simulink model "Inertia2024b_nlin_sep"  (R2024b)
settings: Solver=ode1  StartTime=0.0  StopTime=30  FixedStep=Tstep  EnableMultiTasking=on
model workspace (MAT data in the model file):
  op_snapshot1 : opcond.OperatingPoint (value not decoded)
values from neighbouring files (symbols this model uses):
  T_dis = 2.5    [onebus_nonlinsub.m]
  Ts = Tstep    (= 1e-05)    [onebus_nonlinsub.m]    (also in DemoMTI_Boolean_Index_MTI.m = 1; DemoMTI_EKF.m = 0.02; DemoMTI_MHE_VanDePol.m = 0.01)
  Tstep = 1e-5    (= 1e-05)    [DemoMTI_greyestGFM.m]    (also in onebus_nonlinsub.m)
  Vn = 380    [simulink_parameters_one_bus.m]    (also in nine_bus_parameters.m = 310.*ones(num_inv,1))
  Vtri = Vdc1./3    [simulink_parameters_one_bus.m]    (also in nine_bus_parameters.m = Vdc./2)
  wn = ones(num_inv,1).*w01    [nine_bus_parameters.m]    (also in computeModeFrequencyDampingTable.m = abs(lambda))
undefined symbols (not defined in the file or in its folder): D1_g1, Dsg, Dxd, Dxq, Efdmax_g1, Efdmin_g1, Ibg, K_int_pll, K_prop_pll, KA_g1, kpss_g1, L_1_2, M1_g1, Msg, nom, op, R_1_2, ra_g1, Rsg, T1_g1, T2_g1, T3_g1, T4_g1, TA_g1, Td, Td0p_g1, Tq0p_g1, Tv, Tw_g1, Vbg, xdp_g1, xqp_g1
libraries: spsThreePhaseVIMeasurementLib x5, spsGroundLib x4, slpidlib x4, spsControlledVoltageSourceLib x3, spsControlledCurrentSourceLib x3, spsSeriesRLCBranchLib x3, spsThreePhaseSeriesRLCBranchLib x2, spsThreePhaseSeriesRLCLoadLib x2, spsThreePhaseTransformerTwoWindingsLib x1, spsThreePhaseDynamicLoadLib x1, spsSampleandHoldLib x1, sps_lib x1
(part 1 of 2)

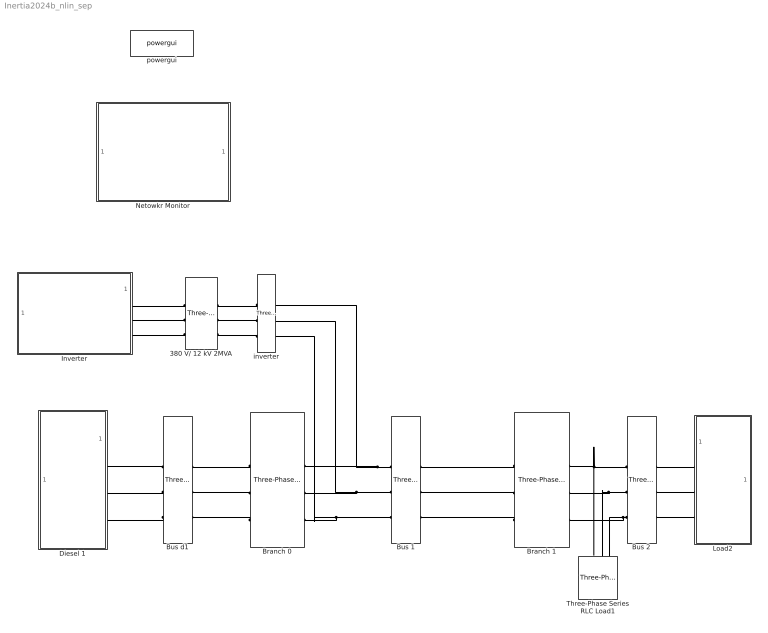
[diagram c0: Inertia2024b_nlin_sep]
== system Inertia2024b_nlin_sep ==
  380 V/ 12 kV 2MVA : spsThreePhaseTransformerTwoWindingsLib/Three-Phase Transformer (Two Windings)  Winding1Connection=Yg  Winding2Connection=Yg  CoreType=Three single-phase transformers  SetSaturation=off  Hysteresis=off  DataFile='hysteresis'  SetInitialFlux=off  Measurements=None  UNITS=pu  NominalPower="[2e6  60]"  Winding1=[12.66e3 , 0.025/30 , 0.025]  Winding2=[380, 0.025/30 , 0.025]  Rm=500  Lm=inf  L0=0.5  Saturation=[ 0,0 ; 0.0024,1.2 ; 1.0,1.52 ]  InitialFluxes=[ 0.8 , -0.8 , 0.7 ]  BreakLoop=off  DiscreteSolver=Trapezoidal iterative  DataType=off  TransfoNumber=0
  Branch 0 : spsThreePhaseSeriesRLCBranchLib/Three-Phase Series RLC Branch  LConnTagsString=A|B|C  RConnTagsString=A|B|C  BranchType=RL  Resistance=0.05  Inductance=0.1/(nom.W)  Capacitance=1e-6  Measurements=None
  Branch 1 : spsThreePhaseSeriesRLCBranchLib/Three-Phase Series RLC Branch  LConnTagsString=A|B|C  RConnTagsString=A|B|C  BranchType=RL  Resistance=R_1_2  Inductance=L_1_2  Capacitance=1e-6  Measurements=None
  Bus 1 : spsThreePhaseVIMeasurementLib/Three-Phase V-I Measurement  VoltageMeasurement=phase-to-ground  SetLabelV=on  LabelV=Vabc1  Vpu=off  VpuLL=off  CurrentMeasurement=yes  SetLabelI=on  LabelI=Iabc1  Ipu=off  Pbase=100e6  Vbase=500e3  OutputType=Complex  PhasorSimulation=off  PSBequivalent=0
  Bus 2 : spsThreePhaseVIMeasurementLib/Three-Phase V-I Measurement  VoltageMeasurement=phase-to-ground  SetLabelV=on  LabelV=Vabc2  Vpu=off  VpuLL=off  CurrentMeasurement=yes  SetLabelI=on  LabelI=Iabc2  Ipu=off  Pbase=100e6  Vbase=500e3  OutputType=Complex  PhasorSimulation=off  PSBequivalent=0
  Bus d1 : spsThreePhaseVIMeasurementLib/Three-Phase V-I Measurement  VoltageMeasurement=phase-to-ground  SetLabelV=on  LabelV=Vabc_d1  Vpu=off  VpuLL=off  CurrentMeasurement=yes  SetLabelI=on  LabelI=Iabc_d1  Ipu=off  Pbase=100e6  Vbase=500e3  OutputType=Complex  PhasorSimulation=off  PSBequivalent=0
  Diesel 1 : Subsystem
  Inverter : Subsystem
  Load2 : Subsystem
  Netowkr Monitor : Subsystem
  Three-Phase Series RLC Load1 : spsThreePhaseSeriesRLCLoadLib/Three-Phase Series RLC Load  LConnTagsString=A|B|C  Configuration=Y (grounded)  NominalVoltage=Vn_pp  Vabc=[1e3 1e3 1e3]  Vabcp=[1e3 1e3 1e3]  NominalFrequency=60  UnbalancedPower=off  ActivePower=P2  InductivePower=Q2  CapacitivePower=0  Pabc=[10e3 9e3 11e3]  QLabc=[100 90 110]  QCabc=[100 90 110]  Pabcp=[10e3 9e3 11e3]  QLabcp=[100 90 110]  QCabcp=[100 90 110]  Measurements=None  LoadType=constant PQ
  inverter : spsThreePhaseVIMeasurementLib/Three-Phase V-I Measurement  VoltageMeasurement=phase-to-ground  SetLabelV=on  LabelV=Vabc_inverter  Vpu=off  VpuLL=off  CurrentMeasurement=yes  SetLabelI=on  LabelI=Iabc_inverter  Ipu=off  Pbase=100e6  Vbase=500e3  OutputType=Complex  PhasorSimulation=off  PSBequivalent=0
  powergui : sps_lib/powergui  Priority=1  SimulationMode=Discrete  SampleTime=Tstep  frequency=60  Iterations=50  frequencyindice=0  Pbase=100e6  ErrMax=1e-4  UnitsV=kV  UnitsW=MW  buscounter=0  FunctionMessages=off  echomessages=off  EnableUseOfTLC=on  CurrentSourceSwitches=off  DisableSnubberDevices=off  DisableRonSwitches=off  DisableVfSwitches=off  DisplayEquations=off  AutomaticDiscreteSolvers=off  SolverType=Tustin/Backward Euler (TBE)  Interpol=off  ExternalGateDelay=off  methode=off  Ts=0  x0status=blocks  SPID=off  SwTol=0  HookPort=off  NonlinearTolerance=1e-4  nMaxIteration=100  ContinueOnMaxIteration=off  RestoreLinks=warning  ResistiveCurrentMeasurement=off  Frange=[0:2:500]  Ylog=off  Xlog=on  ShowGrid=off  save=off  variable=ZData  structure=0  ZoomFFT=on  StartTime=0.0  cycles=1  DisplayStyle=1  fundamental=60  FreqAxis=off  MaxFrequency=1000  frequencyindicesteady=1  RmsSteady=1  display=off
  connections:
  Branch 1/LConn1 -- Bus 1/RConn1
  Branch 1/LConn2 -- Bus 1/RConn2
  Branch 1/LConn3 -- Bus 1/RConn3
  Bus 2/LConn1 -- Three-Phase Series RLC Load1/LConn1 -- Branch 1/RConn1
  Bus 2/LConn2 -- Three-Phase Series RLC Load1/LConn2 -- Branch 1/RConn2
  Bus 2/LConn3 -- Three-Phase Series RLC Load1/LConn3 -- Branch 1/RConn3
  Bus 1/LConn1 -- inverter/RConn1 -- Branch 0/RConn1
  Bus 1/LConn2 -- inverter/RConn2 -- Branch 0/RConn2
  Bus 1/LConn3 -- inverter/RConn3 -- Branch 0/RConn3
  Branch 0/LConn1 -- Bus d1/RConn1
  Bus d1/LConn1 -- Diesel 1/RConn1
  Branch 0/LConn3 -- Bus d1/RConn3
  Bus d1/LConn3 -- Diesel 1/RConn3
  Bus d1/LConn2 -- Diesel 1/RConn2
  Branch 0/LConn2 -- Bus d1/RConn2
  Bus 2/RConn3 -- Load2/LConn3
  Bus 2/RConn2 -- Load2/LConn2
  Bus 2/RConn1 -- Load2/LConn1
  Inverter/RConn2 -- 380 V/ 12 kV 2MVA/RConn2
  inverter/LConn2 -- 380 V/ 12 kV 2MVA/LConn2
  inverter/LConn1 -- 380 V/ 12 kV 2MVA/LConn1
  Inverter/RConn1 -- 380 V/ 12 kV 2MVA/RConn1
  Inverter/RConn3 -- 380 V/ 12 kV 2MVA/RConn3
  inverter/LConn3 -- 380 V/ 12 kV 2MVA/LConn3

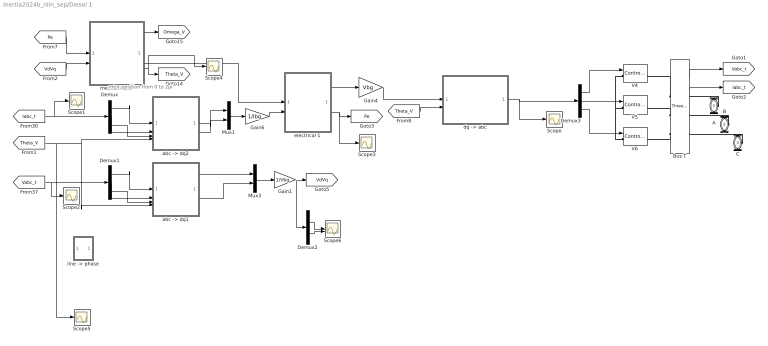
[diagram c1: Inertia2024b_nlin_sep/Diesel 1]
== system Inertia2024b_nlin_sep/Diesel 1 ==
  note: rotor position from 0 to 2pi
  Bus T : spsThreePhaseVIMeasurementLib/Three-Phase V-I Measurement  VoltageMeasurement=phase-to-ground  SetLabelV=off  LabelV=Vabc_d1  Vpu=off  VpuLL=off  CurrentMeasurement=yes  SetLabelI=off  LabelI=Iabc_d1  Ipu=off  Pbase=100e6  Vbase=500e3  OutputType=Complex  PhasorSimulation=off  PSBequivalent=0
  Demux : Demux  Outputs=3
  Demux1 : Demux  Outputs=3
  Demux2 : Demux  Outputs=2
  Demux3 : Demux  Outputs=3
  Gain1 : Gain  Gain=1/Vbg
  Gain4 : Gain  Gain=Vbg
  Gain6 : Gain  Gain=1/Ibg
  Mux1 : Mux  Inputs=2
  Mux3 : Mux  Inputs=2
  Scope{,1..5} (6 alike) : Scope
  Scope6 : Scope  NumInputPorts=2
  V4 : spsControlledVoltageSourceLib/Controlled Voltage Source  Initialize=off  Source_Type=AC  Amplitude=Vbg  Phase=0  Frequency=60  Measurements=None
  V5 : spsControlledVoltageSourceLib/Controlled Voltage Source  Initialize=off  Source_Type=AC  Amplitude=Vbg  Phase=-120  Frequency=60  Measurements=None
  V6 : spsControlledVoltageSourceLib/Controlled Voltage Source  Initialize=off  Source_Type=AC  Amplitude=Vbg  Phase=120  Frequency=60  Measurements=None
  "abc -> dq1" : Subsystem
  "abc -> dq2" : Subsystem
  "dq -> abc" : Subsystem
  electrical 1 : Subsystem
  "line -> phase" : Subsystem  Commented=on
  mechanical 1 : Subsystem
  A : PMIOPort  Side=Right
  B : PMIOPort  Port=2  Side=Right
  C : PMIOPort  Port=3  Side=Right
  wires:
  "abc -> dq2"/1(d) -> Mux1/1
  "abc -> dq1"/1(d) -> Mux3/1
  [Theta_V] -> Scope5/1, "abc -> dq2"/4(Theta), "abc -> dq1"/4(Theta)
  "abc -> dq2"/2(q) -> Mux1/2
  Mux1/1 -> Gain6/1
  electrical 1/2(Pe) -> Scope3/1, [Pe]
  mechanical 1/2(Ef) -> electrical 1/1(Efd)
  electrical 1/1(VdVqref) -> Gain4/1
  Gain6/1 -> electrical 1/2(IdIq)
  Gain4/1 -> "dq -> abc"/1(dq)
  [Theta_V] -> "dq -> abc"/2(Theta)
  Mux3/1 -> Gain1/1
  Gain1/1 -> Demux2/1, [VdVq]
  Demux3/1 -> V4/1
  Demux3/2 -> V5/1
  Demux3/3 -> V6/1
  "dq -> abc"/1(abc) -> Demux3/1, Scope/1
  [Iabc_t] -> Scope1/1, Demux/1
  Demux/1 -> "abc -> dq2"/1(a)
  Demux/2 -> "abc -> dq2"/2(b)
  Demux/3 -> "abc -> dq2"/3(c)
  "abc -> dq1"/2(q) -> Mux3/2
  Demux1/2 -> "abc -> dq1"/2(b)
  Demux1/1 -> "abc -> dq1"/1(a)
  Demux1/3 -> "abc -> dq1"/3(c)
  [Vabc_t] -> Scope2/1, Demux1/1
  mechanical 1/1(w) -> [Omega_V]
  [Pe] -> mechanical 1/1(Pe)
  [VdVq] -> mechanical 1/2(VdVqFB)
  Bus T/1 -> [Vabc_t]
  Bus T/2 -> [Iabc_t]
  mechanical 1/3(rotor angle) -> Scope4/1, [Theta_V]
  Demux2/1 -> Scope6/1
  Demux2/2 -> Scope6/2
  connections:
  V5/LConn1 -- V4/LConn1 -- V6/LConn1
  Bus T/LConn1 -- V4/RConn1
  Bus T/LConn2 -- V5/RConn1
  Bus T/LConn3 -- V6/RConn1
  C/RConn1 -- Bus T/RConn3
  B/RConn1 -- Bus T/RConn2
  A/RConn1 -- Bus T/RConn1

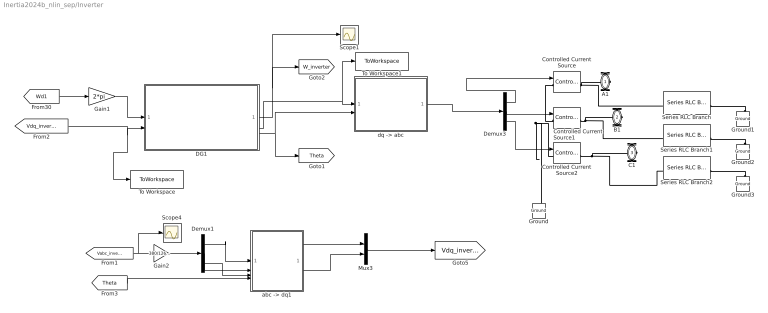
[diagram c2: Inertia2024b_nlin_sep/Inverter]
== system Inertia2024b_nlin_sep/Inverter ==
  Controlled Current Source : spsControlledCurrentSourceLib/Controlled Current Source  Initialize=off  Source_Type=AC  Amplitude=0  Phase=0  Frequency=0  Measurements=None
  Controlled Current Source1 : spsControlledCurrentSourceLib/Controlled Current Source  Initialize=off  Source_Type=AC  Amplitude=0  Phase=0  Frequency=0  Measurements=None
  Controlled Current Source2 : spsControlledCurrentSourceLib/Controlled Current Source  Initialize=off  Source_Type=AC  Amplitude=0  Phase=0  Frequency=0  Measurements=None
  DG1 : Subsystem  ReferencedSubsystem=inverter_nonlinear_model2024b  rdc=rdc1  Ldc=Ldc1  Cdc=Cdc1  Vdc=Vdc1  Cf=Cf1  Lf=Lf1  rf=rf1  rc=rc1  Lc=Lc1  wc=wc1  mp=mp1  nq=nq1  Vn=Vn(1)  wn=wn(1)  Kic=Kic1  Kpc=Kpc1  Kiv=Kiv1  Kpv=Kpv1  F=F1  Vtri=Vtri(1)  x0=x01
  Demux1 : Demux  Outputs=3
  Demux3 : Demux  Outputs=3
  Gain1 : Gain  Gain=2*pi
  Gain2 : Gain  Gain=380/12600
  Ground{,1..3} (4 alike) : spsGroundLib/Ground  LConnTagsString=a
  Mux3 : Mux  Inputs=2
  Scope1 : Scope
  Scope4 : Scope
  Series RLC Branch : spsSeriesRLCBranchLib/Series RLC Branch  LConnTagsString=__new0  RConnTagsString=__new0  BranchType=RLC  Resistance=1e6  Inductance=0  SetiL0=off  InitialCurrent=0  Capacitance=0  Setx0=off  InitialVoltage=0  Measurements=None
  Series RLC Branch1 : spsSeriesRLCBranchLib/Series RLC Branch  LConnTagsString=__new0  RConnTagsString=__new0  BranchType=RLC  Resistance=1e6  Inductance=0  SetiL0=off  InitialCurrent=0  Capacitance=0  Setx0=off  InitialVoltage=0  Measurements=None
  Series RLC Branch2 : spsSeriesRLCBranchLib/Series RLC Branch  LConnTagsString=__new0  RConnTagsString=__new0  BranchType=RLC  Resistance=1e6  Inductance=0  SetiL0=off  InitialCurrent=0  Capacitance=0  Setx0=off  InitialVoltage=0  Measurements=None
  To Workspace : ToWorkspace  VariableName=Vdq_inv  SaveFormat=Timeseries  SampleTime=-1
  To Workspace1 : ToWorkspace  VariableName=ioDQ  SaveFormat=Timeseries  SampleTime=-1
  "abc -> dq1" : Subsystem
  "dq -> abc" : Subsystem
  A1 : PMIOPort  Side=Right
  B1 : PMIOPort  Port=2  Side=Right
  C1 : PMIOPort  Port=3  Side=Right
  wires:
  [Wd1] -> Gain1/1
  DG1/2 -> To Workspace1/1, "dq -> abc"/1(dq)
  "dq -> abc"/1(abc) -> Demux3/1
  Demux3/3 -> Controlled Current Source2/1
  Demux3/2 -> Controlled Current Source1/1
  Demux3/1 -> Controlled Current Source/1
  Gain1/1 -> DG1/1
  [Vdq_inverter] -> To Workspace/1, DG1/2
  Demux1/2 -> "abc -> dq1"/2(b)
  "abc -> dq1"/1(d) -> Mux3/1
  [Theta] -> "abc -> dq1"/4(Theta)
  [Vabc_inverter] -> Scope4/1, Gain2/1
  Mux3/1 -> [Vdq_inverter]
  "abc -> dq1"/2(q) -> Mux3/2
  Demux1/1 -> "abc -> dq1"/1(a)
  Demux1/3 -> "abc -> dq1"/3(c)
  DG1/3 -> "dq -> abc"/2(Theta), [Theta]
  DG1/1 -> [W_inverter], Scope1/1
  Gain2/1 -> Demux1/1
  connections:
  Controlled Current Source/LConn1 -- Ground/LConn1 -- Controlled Current Source2/LConn1 -- Controlled Current Source1/LConn1
  Controlled Current Source/RConn1 -- Series RLC Branch/LConn1 -- A1/RConn1
  Controlled Current Source1/RConn1 -- Series RLC Branch1/LConn1 -- B1/RConn1
  Controlled Current Source2/RConn1 -- Series RLC Branch2/LConn1 -- C1/RConn1
  Ground1/LConn1 -- Series RLC Branch/RConn1
  Ground2/LConn1 -- Series RLC Branch1/RConn1
  Ground3/LConn1 -- Series RLC Branch2/RConn1

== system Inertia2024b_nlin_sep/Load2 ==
  Bus Selector2 : BusSelector  OutputSignals=Positive-sequence voltage V (pu),Active power P (W),Reactive power Q (var)
  P3 : spsThreePhaseDynamicLoadLib/Three-Phase Dynamic Load  NominalVoltage=[nom.V nom.F]  ActiveReactivePowers="[op.PL1  op.QL1]"  PositiveSequence=[1 0]  ExternalControl=on  NpNq=[0 0]  TimeConstants="[0  0  0  0]"  MinimumVoltage=0.7  Tfilter=1e-4  LoadFlowParameters=[4,0,0,0,0]
  PQref3 : Subsystem
  Three-Phase Series RLC Load : spsThreePhaseSeriesRLCLoadLib/Three-Phase Series RLC Load  LConnTagsString=A|B|C  Configuration=Y (grounded)  NominalVoltage=nom.V  Vabc=[1e3 1e3 1e3]  Vabcp=[1e3 1e3 1e3]  NominalFrequency=nom.F  UnbalancedPower=off  ActivePower=10e3  InductivePower=0  CapacitivePower=0  Pabc=[10e3 9e3 11e3]  QLabc=[100 90 110]  QCabc=[100 90 110]  Pabcp=[10e3 9e3 11e3]  QLabcp=[100 90 110]  QCabcp=[100 90 110]  Measurements=None  LoadType=constant PQ
  scope7 : Scope
  A : PMIOPort  Side=Left
  B : PMIOPort  Port=2  Side=Left
  C : PMIOPort  Port=3  Side=Left
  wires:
  P3/1 -> scope7/1, Bus Selector2/1
  Bus Selector2/1 -> PQref3/1(V), [V_Load10]  "<Positive-sequence voltage V (pu)>"
  Bus Selector2/2 -> [P_Load10]  "<Active power P (W)>"
  Bus Selector2/3 -> [Q_Load10]  "<Reactive power Q (var)>"
  PQref3/1(PQ) -> P3/1
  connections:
  C/RConn1 -- Three-Phase Series RLC Load/LConn3 -- P3/LConn3
  B/RConn1 -- Three-Phase Series RLC Load/LConn2 -- P3/LConn2
  A/RConn1 -- Three-Phase Series RLC Load/LConn1 -- P3/LConn1

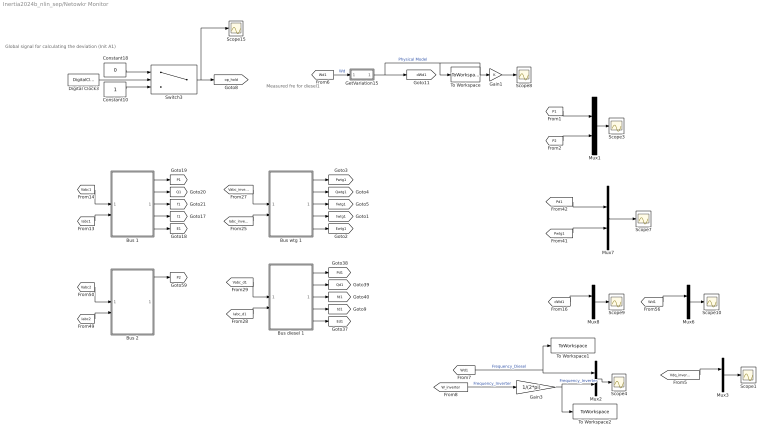
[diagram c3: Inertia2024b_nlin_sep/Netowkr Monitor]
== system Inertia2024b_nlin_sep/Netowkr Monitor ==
  note: Global signal for calculating the deviation (Init A1)
  note: Measured fre for diesel1
  Bus 1 : Subsystem
  Bus 2 : Subsystem
  Bus diesel 1 : Subsystem
  Bus wtg 1 : Subsystem
  Constant10 : Constant
  Constant18 : Constant  Value=0
  Digital Clock3 : DigitalClock  SampleTime=Ts
  Gain1 : Gain
  Gain3 : Gain  Gain=1/(2*pi)
  GetVariation15 : Subsystem
  Mux1 : Mux  Inputs=2
  Mux2 : Mux  Inputs=2
  Mux3 : Mux  Inputs=1
  Mux6 : Mux  Inputs=1
  Mux7 : Mux  Inputs=2
  Mux8 : Mux  Inputs=1
  Scope{1,3..4,7..10,15} (8 alike) : Scope
  Switch3 : Switch  Threshold=T_dis
  To Workspace : ToWorkspace  VariableName=y_con  SaveFormat=Structure With Time  SampleTime=-1
  To Workspace1 : ToWorkspace  VariableName=Wd1  SaveFormat=Timeseries  SampleTime=-1
  To Workspace2 : ToWorkspace  VariableName=W_inverter  SaveFormat=Timeseries  SampleTime=-1
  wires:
  [Vabc1] -> Bus 1/1(Vabc)
  [Iabc1] -> Bus 1/2(I_abc)
  Bus 1/1(P_meas) -> [P1]
  Bus 1/2(Q_meas) -> [Q1]
  Bus 1/3(w_meas) -> [f1]
  Bus 1/4(theta) -> [t1]
  Bus 1/5(E) -> [E1]
  Mux1/1 -> Scope3/1
  [P2] -> Mux1/2
  [P1] -> Mux1/1
  [Vabc_inverter] -> Bus wtg 1/1(Vabc)
  [Iabc_inverter] -> Bus wtg 1/2(I_abc)
  Bus wtg 1/1(P_meas) -> [Pwtg1]
  Bus wtg 1/2(Q_meas) -> [Qwtg1]
  Bus wtg 1/3(w_meas) -> [fwtg1]
  Bus wtg 1/4(theta) -> [twtg1]
  Bus wtg 1/5(E) -> [Ewtg1]
  [Pd1] -> Mux7/1
  Mux7/1 -> Scope7/1
  [Pwtg1] -> Mux7/2
  [Vabc2] -> Bus 2/1(Vabc)
  [Iabc2] -> Bus 2/2(I_abc)
  Bus 2/1(P_meas) -> [P2]
  [Wd1] -> Mux6/1
  Mux6/1 -> Scope10/1
  Switch3/1 -> [op_hold], Scope15/1
  Constant10/1 -> Switch3/3
  Digital Clock3/1 -> Switch3/2
  Constant18/1 -> Switch3/1
  [Wd1] -> GetVariation15/1(In1)  "Wd"
  GetVariation15/1(Out1) -> Gain1/1, To Workspace/1, [dWd1]  "Physical Model"
  Gain1/1 -> Scope8/1
  Mux8/1 -> Scope9/1
  [dWd1] -> Mux8/1
  Bus diesel 1/4(theta) -> [td1]
  Bus diesel 1/3(w_meas) -> [fd1]
  [Vabc_d1] -> Bus diesel 1/1(Vabc)
  Bus diesel 1/5(E) -> [Ed1]
  Bus diesel 1/2(Q_meas) -> [Qd1]
  [Iabc_d1] -> Bus diesel 1/2(I_abc)
  Bus diesel 1/1(P_meas) -> [Pd1]
  Mux3/1 -> Scope1/1
  [Vdq_inverter] -> Mux3/1
  Gain3/1 -> To Workspace2/1, Mux2/2  "Frequency_Inverter"
  [W_inverter] -> Gain3/1  "Frequency_Inverter"
  [Wd1] -> To Workspace1/1, Mux2/1  "Frequency_Diesel"
  Mux2/1 -> Scope4/1

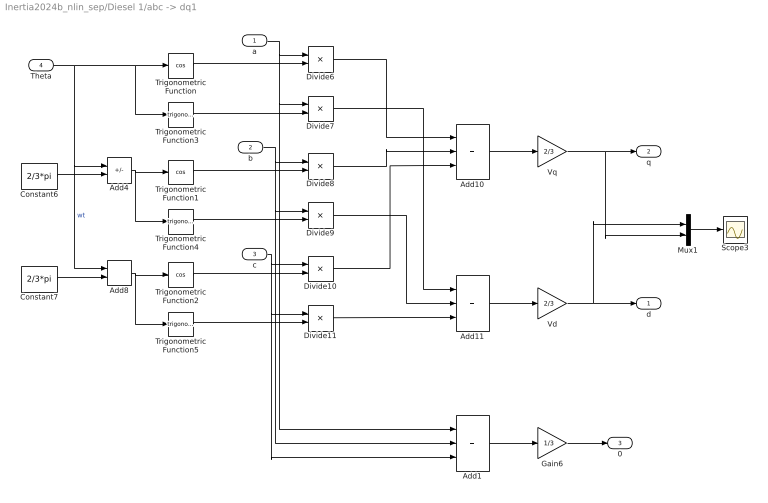
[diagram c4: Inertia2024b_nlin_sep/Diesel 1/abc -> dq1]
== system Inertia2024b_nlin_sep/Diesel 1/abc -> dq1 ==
  a : Inport
  b : Inport  Port=2
  c : Inport  Port=3
  Theta : Inport  Port=4
  Add1 : Sum  Inputs=+++
  Add10 : Sum  Inputs=+++
  Add11 : Sum  Inputs=+++
  Add4 : Sum  Inputs=+-
  Add8 : Sum
  Constant6 : Constant  Value=2/3*pi
  Constant7 : Constant  Value=2/3*pi
  Divide{6..11} (6 alike) : Product  Inputs=**
  Gain6 : Gain  Gain=1/3
  Mux1 : Mux  Inputs=2
  Scope3 : Scope
  Trigonometric Function : Trigonometry  Operator=cos
  Trigonometric Function1 : Trigonometry  Operator=cos
  Trigonometric Function2 : Trigonometry  Operator=cos
  Trigonometric Function3 : Trigonometry
  Trigonometric Function4 : Trigonometry
  Trigonometric Function5 : Trigonometry
  Vd : Gain  Gain=2/3
  Vq : Gain  Gain=2/3
  d : Outport  VectorParamsAs1DForOutWhenUnconnected=off
  q : Outport  Port=2  VectorParamsAs1DForOutWhenUnconnected=off
  0 : Outport  Port=3  VectorParamsAs1DForOutWhenUnconnected=off
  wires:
  Theta/1 -> Add4/1, Add8/1, Trigonometric Function/1, Trigonometric Function3/1  "wt"
  Constant6/1 -> Add4/2
  Add4/1 -> Trigonometric Function1/1, Trigonometric Function4/1
  Add8/1 -> Trigonometric Function2/1, Trigonometric Function5/1
  Trigonometric Function3/1 -> Divide7/2
  Trigonometric Function4/1 -> Divide9/2
  Trigonometric Function5/1 -> Divide11/2
  a/1 -> Divide6/1, Divide7/1, Add1/1
  Trigonometric Function/1 -> Divide6/2
  Trigonometric Function2/1 -> Divide10/2
  Trigonometric Function1/1 -> Divide8/2
  b/1 -> Divide8/1, Divide9/1, Add1/2
  c/1 -> Divide10/1, Divide11/1, Add1/3
  Constant7/1 -> Add8/2
  Divide6/1 -> Add10/1
  Divide8/1 -> Add10/2
  Divide10/1 -> Add10/3
  Divide7/1 -> Add11/1
  Divide9/1 -> Add11/2
  Divide11/1 -> Add11/3
  Add10/1 -> Vq/1
  Add11/1 -> Vd/1
  Vq/1 -> Mux1/2, q/1
  Vd/1 -> Mux1/1, d/1
  Add1/1 -> Gain6/1
  Gain6/1 -> 0/1
  Mux1/1 -> Scope3/1

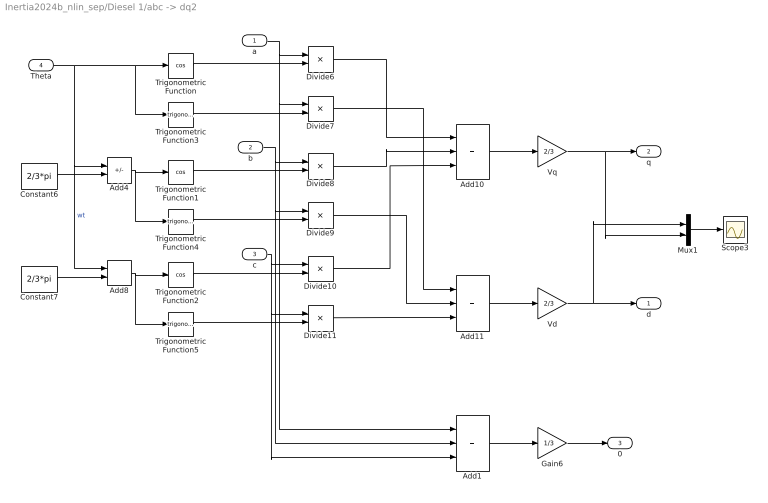
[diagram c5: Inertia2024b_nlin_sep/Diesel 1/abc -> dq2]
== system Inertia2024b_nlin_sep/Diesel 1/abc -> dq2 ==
  a : Inport
  b : Inport  Port=2
  c : Inport  Port=3
  Theta : Inport  Port=4
  Add1 : Sum  Inputs=+++
  Add10 : Sum  Inputs=+++
  Add11 : Sum  Inputs=+++
  Add4 : Sum  Inputs=+-
  Add8 : Sum
  Constant6 : Constant  Value=2/3*pi
  Constant7 : Constant  Value=2/3*pi
  Divide{6..11} (6 alike) : Product  Inputs=**
  Gain6 : Gain  Gain=1/3
  Mux1 : Mux  Inputs=2
  Scope3 : Scope
  Trigonometric Function : Trigonometry  Operator=cos
  Trigonometric Function1 : Trigonometry  Operator=cos
  Trigonometric Function2 : Trigonometry  Operator=cos
  Trigonometric Function3 : Trigonometry
  Trigonometric Function4 : Trigonometry
  Trigonometric Function5 : Trigonometry
  Vd : Gain  Gain=2/3
  Vq : Gain  Gain=2/3
  d : Outport  VectorParamsAs1DForOutWhenUnconnected=off
  q : Outport  Port=2  VectorParamsAs1DForOutWhenUnconnected=off
  0 : Outport  Port=3  VectorParamsAs1DForOutWhenUnconnected=off
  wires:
  Theta/1 -> Add4/1, Add8/1, Trigonometric Function/1, Trigonometric Function3/1  "wt"
  Constant6/1 -> Add4/2
  Add4/1 -> Trigonometric Function1/1, Trigonometric Function4/1
  Add8/1 -> Trigonometric Function2/1, Trigonometric Function5/1
  Trigonometric Function3/1 -> Divide7/2
  Trigonometric Function4/1 -> Divide9/2
  Trigonometric Function5/1 -> Divide11/2
  a/1 -> Divide6/1, Divide7/1, Add1/1
  Trigonometric Function/1 -> Divide6/2
  Trigonometric Function2/1 -> Divide10/2
  Trigonometric Function1/1 -> Divide8/2
  b/1 -> Divide8/1, Divide9/1, Add1/2
  c/1 -> Divide10/1, Divide11/1, Add1/3
  Constant7/1 -> Add8/2
  Divide6/1 -> Add10/1
  Divide8/1 -> Add10/2
  Divide10/1 -> Add10/3
  Divide7/1 -> Add11/1
  Divide9/1 -> Add11/2
  Divide11/1 -> Add11/3
  Add10/1 -> Vq/1
  Add11/1 -> Vd/1
  Vq/1 -> Mux1/2, q/1
  Vd/1 -> Mux1/1, d/1
  Add1/1 -> Gain6/1
  Gain6/1 -> 0/1
  Mux1/1 -> Scope3/1

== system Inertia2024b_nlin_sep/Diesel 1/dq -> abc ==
  dq : Inport
  Theta : Inport  Port=2
  Demux : Demux  Outputs=2
  Mux : Mux  Inputs=3
  Transport Delay : TransportDelay  DelayTime=1e-4
  "dq -> abc1" : Subsystem
  abc : Outport  VectorParamsAs1DForOutWhenUnconnected=off
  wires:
  "dq -> abc1"/1(a) -> Mux/1
  "dq -> abc1"/2(b) -> Mux/2
  "dq -> abc1"/3(c) -> Mux/3
  Mux/1 -> Transport Delay/1
  Theta/1 -> "dq -> abc1"/3(Theta)
  dq/1 -> Demux/1
  Transport Delay/1 -> abc/1
  Demux/1 -> "dq -> abc1"/1(d)
  Demux/2 -> "dq -> abc1"/2(q)

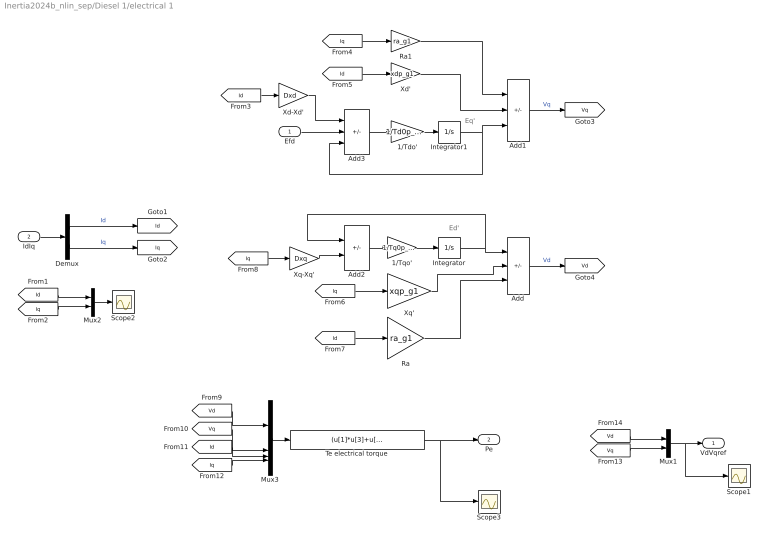
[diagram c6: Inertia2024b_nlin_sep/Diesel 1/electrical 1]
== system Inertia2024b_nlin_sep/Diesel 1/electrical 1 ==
  note: Ed'
  note: Eq'
  Efd : Inport
  IdIq : Inport  Port=2
  1/Tdo' : Gain  Gain=1/Td0p_g1
  1/Tqo' : Gain  Gain=1/Tq0p_g1
  Add : Sum  Inputs=++-
  Add1 : Sum  Inputs=--+
  Add2 : Sum  Inputs=-+
  Add3 : Sum  Inputs=-+-
  Demux : Demux  Outputs=2
  Integrator : Integrator  IgnoreLimit=on
  Integrator1 : Integrator  InitialCondition=1  IgnoreLimit=on
  Mux1 : Mux  Inputs=2
  Mux2 : Mux  Inputs=2
  Mux3 : Mux
  Ra : Gain  Gain=ra_g1
  Ra1 : Gain  Gain=ra_g1
  Scope1 : Scope
  Scope2 : Scope
  Scope3 : Scope
  Te electrical torque : Fcn  Expr=(u[1]*u[3]+u[2]*u[4])
  Xd' : Gain  Gain=xdp_g1
  Xd-Xd' : Gain  Gain=Dxd
  Xq' : Gain  Gain=xqp_g1
  Xq-Xq' : Gain  Gain=Dxq
  VdVqref : Outport  VectorParamsAs1DForOutWhenUnconnected=off
  Pe : Outport  Port=2  VectorParamsAs1DForOutWhenUnconnected=off
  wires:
  Mux1/1 -> Scope1/1, VdVqref/1
  1/Tqo'/1 -> Integrator/1
  Add2/1 -> 1/Tqo'/1
  Integrator/1 -> Add2/1, Add/1
  Xq'/1 -> Add/2
  Xq-Xq'/1 -> Add2/2
  Demux/2 -> [Iq]  "Iq"
  1/Tdo'/1 -> Integrator1/1
  Add3/1 -> 1/Tdo'/1
  Integrator1/1 -> Add1/3, Add3/3
  Efd/1 -> Add3/2
  Xd-Xd'/1 -> Add3/1
  Demux/1 -> [Id]  "Id"
  Mux3/1 -> Te electrical torque/1
  IdIq/1 -> Demux/1
  Te electrical torque/1 -> Scope3/1, Pe/1
  Mux2/1 -> Scope2/1
  Ra/1 -> Add/3
  Xd'/1 -> Add1/2
  Ra1/1 -> Add1/1
  [Iq] -> Mux2/2
  [Id] -> Mux2/1
  Add1/1 -> [Vq]  "Vq"
  Add/1 -> [Vd]  "Vd"
  [Id] -> Xd-Xd'/1
  [Iq] -> Ra1/1
  [Id] -> Xd'/1
  [Iq] -> Xq'/1
  [Id] -> Ra/1
  [Iq] -> Xq-Xq'/1
  [Vd] -> Mux3/1
  [Vq] -> Mux3/2
  [Id] -> Mux3/3
  [Iq] -> Mux3/4
  [Vd] -> Mux1/1
  [Vq] -> Mux1/2

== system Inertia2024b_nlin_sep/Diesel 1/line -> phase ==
  Vll : Inport
  Add1 : Sum  Inputs=+-
  Add2 : Sum  Inputs=+-
  Add3 : Sum  Inputs=+-
  Demux1 : Demux  Outputs=3
  Gain : Gain  Gain=1/3
  Mux : Mux  Inputs=3
  Vph : Outport  VectorParamsAs1DForOutWhenUnconnected=off
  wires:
  Demux1/1 -> Add1/1, Add2/2
  Demux1/3 -> Add1/2, Add3/1
  Demux1/2 -> Add2/1, Add3/2
  Add1/1 -> Mux/1
  Add2/1 -> Mux/2
  Add3/1 -> Mux/3
  Vll/1 -> Demux1/1
  Mux/1 -> Gain/1
  Gain/1 -> Vph/1

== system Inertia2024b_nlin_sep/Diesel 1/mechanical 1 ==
  Pe : Inport
  VdVqFB : Inport  Port=2
  Add1 : Sum
  Add2 : Sum
  Constant1 : Constant  Value=1.037
  Constant2 : Constant
  Constant3 : Constant  Value=377
  Constant4 : Constant  Value=2*pi
  Demux : Demux  Outputs=2
  Exciter : Subsystem
  Gain : Gain  Gain=2*pi
  Gain1 : Gain  Gain=1/(2*pi)
  Integrator : Integrator  InitialCondition=2*pi*60  ZeroCross=off
  Math Function : Math  Operator=square  SignedPower=on
  Math Function1 : Math  Operator=square  SignedPower=on
  Math Function2 : Math  Operator=mod  SignedPower=on
  PSS : Subsystem
  Saturation : Saturate  UpperLimit=0.15  LowerLimit=-0.15
  Scope{1..5} (5 alike) : Scope
  Sqrt : Sqrt
  thermal_turbine_droop1 : Subsystem
  w : Outport  VectorParamsAs1DForOutWhenUnconnected=off
  Ef : Outport  Port=2  VectorParamsAs1DForOutWhenUnconnected=off
  rotor angle : Outport  Port=3  VectorParamsAs1DForOutWhenUnconnected=off
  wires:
  thermal_turbine_droop1/1(dww) -> [dww], Scope2/1, Add1/1, PSS/1(dw), thermal_turbine_droop1/1(dw)
  Integrator/1 -> Gain/1
  Gain/1 -> Math Function2/1
  Math Function2/1 -> rotor angle/1
  Constant4/1 -> Math Function2/2
  Constant3/1 -> Add1/2
  Constant1/1 -> Exciter/2(Vtr0)
  Add2/1 -> Sqrt/1
  Math Function1/1 -> Add2/2
  Math Function/1 -> Add2/1
  Sqrt/1 -> Exciter/1(Vt)
  Demux/1 -> Math Function/1
  Demux/2 -> Math Function1/1
  VdVqFB/1 -> Demux/1
  Pe/1 -> thermal_turbine_droop1/2(pe)
  PSS/1(Vpss) -> Scope3/1, Saturation/1
  Saturation/1 -> Scope4/1, Exciter/3(Vpss)
  Exciter/1(Ef) -> Scope5/1, Ef/1
  Add1/1 -> Gain1/1
  Gain1/1 -> Scope1/1, [Wd1], w/1, Integrator/1

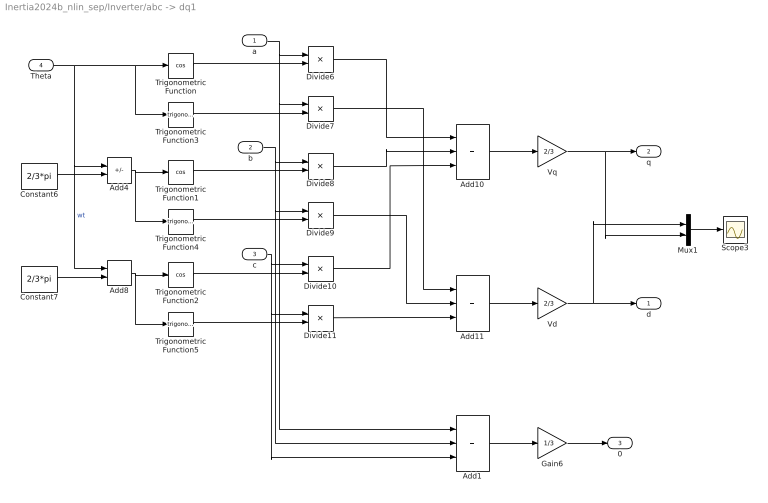
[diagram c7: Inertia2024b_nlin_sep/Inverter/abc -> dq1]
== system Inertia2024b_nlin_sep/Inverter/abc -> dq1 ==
  a : Inport
  b : Inport  Port=2
  c : Inport  Port=3
  Theta : Inport  Port=4
  Add1 : Sum  Inputs=+++
  Add10 : Sum  Inputs=+++
  Add11 : Sum  Inputs=+++
  Add4 : Sum  Inputs=+-
  Add8 : Sum
  Constant6 : Constant  Value=2/3*pi
  Constant7 : Constant  Value=2/3*pi
  Divide{6..11} (6 alike) : Product  Inputs=**
  Gain6 : Gain  Gain=1/3
  Mux1 : Mux  Inputs=2
  Scope3 : Scope
  Trigonometric Function : Trigonometry  Operator=cos
  Trigonometric Function1 : Trigonometry  Operator=cos
  Trigonometric Function2 : Trigonometry  Operator=cos
  Trigonometric Function3 : Trigonometry
  Trigonometric Function4 : Trigonometry
  Trigonometric Function5 : Trigonometry
  Vd : Gain  Gain=2/3
  Vq : Gain  Gain=2/3
  d : Outport  VectorParamsAs1DForOutWhenUnconnected=off
  q : Outport  Port=2  VectorParamsAs1DForOutWhenUnconnected=off
  0 : Outport  Port=3  VectorParamsAs1DForOutWhenUnconnected=off
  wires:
  Theta/1 -> Add4/1, Add8/1, Trigonometric Function/1, Trigonometric Function3/1  "wt"
  Constant6/1 -> Add4/2
  Add4/1 -> Trigonometric Function1/1, Trigonometric Function4/1
  Add8/1 -> Trigonometric Function2/1, Trigonometric Function5/1
  Trigonometric Function3/1 -> Divide7/2
  Trigonometric Function4/1 -> Divide9/2
  Trigonometric Function5/1 -> Divide11/2
  a/1 -> Divide6/1, Divide7/1, Add1/1
  Trigonometric Function/1 -> Divide6/2
  Trigonometric Function2/1 -> Divide10/2
  Trigonometric Function1/1 -> Divide8/2
  b/1 -> Divide8/1, Divide9/1, Add1/2
  c/1 -> Divide10/1, Divide11/1, Add1/3
  Constant7/1 -> Add8/2
  Divide6/1 -> Add10/1
  Divide8/1 -> Add10/2
  Divide10/1 -> Add10/3
  Divide7/1 -> Add11/1
  Divide9/1 -> Add11/2
  Divide11/1 -> Add11/3
  Add10/1 -> Vq/1
  Add11/1 -> Vd/1
  Vq/1 -> Mux1/2, q/1
  Vd/1 -> Mux1/1, d/1
  Add1/1 -> Gain6/1
  Gain6/1 -> 0/1
  Mux1/1 -> Scope3/1

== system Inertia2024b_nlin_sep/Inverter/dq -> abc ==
  dq : Inport
  Theta : Inport  Port=2
  Demux : Demux  Outputs=2
  Mux : Mux  Inputs=3
  "dq -> abc1" : Subsystem
  abc : Outport  VectorParamsAs1DForOutWhenUnconnected=off
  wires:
  "dq -> abc1"/1(a) -> Mux/1
  "dq -> abc1"/2(b) -> Mux/2
  "dq -> abc1"/3(c) -> Mux/3
  Theta/1 -> "dq -> abc1"/3(Theta)
  dq/1 -> Demux/1
  Demux/1 -> "dq -> abc1"/1(d)
  Demux/2 -> "dq -> abc1"/2(q)
  Mux/1 -> abc/1

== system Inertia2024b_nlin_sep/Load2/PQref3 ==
  V : Inport
  Add1 : Sum  Inputs=+++
  Add2 : Sum  Inputs=+++
  Bus Selector : BusSelector  OutputSignals=Positive-sequence voltage V (pu)
  Constant : Constant  Value=op.PL1+op.PL1_dis
  Constant1 : Constant  Value=op.QL1
  Constant2 : Constant  Value=op.PL1
  Digital Clock : DigitalClock  SampleTime=Ts
  I : Gain  Gain=0.1
  I1 : Gain  Gain=0.1
  Mux : Mux  Inputs=2
  P : Gain  Gain=0.8
  P1 : Gain  Gain=0.8
  Product : Product  Inputs=3  RndMeth=Zero
  Product1 : Product  RndMeth=Zero
  Product2 : Product  Inputs=3  RndMeth=Zero
  Product3 : Product  RndMeth=Zero
  Switch : Switch  Threshold=T_dis
  Z : Gain  Gain=0.1
  Z1 : Gain  Gain=0.1
  scope7 : Scope
  PQ : Outport  VectorParamsAs1DForOutWhenUnconnected=off
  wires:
  V/1 -> Bus Selector/1
  Product/1 -> Z/1
  Bus Selector/1 -> scope7/1, Product/2, Product/3, Product1/2, Product2/2, Product2/3, Product3/2  "<Positive-sequence voltage V (pu)>"
  Z/1 -> Add1/1
  Product1/1 -> I/1
  I/1 -> Add1/2
  P/1 -> Add1/3
  Mux/1 -> PQ/1
  Product2/1 -> Z1/1
  Z1/1 -> Add2/1
  Product3/1 -> I1/1
  I1/1 -> Add2/2
  P1/1 -> Add2/3
  Add1/1 -> Mux/1
  Add2/1 -> Mux/2
  Constant1/1 -> Product2/1, Product3/1, P1/1
  Digital Clock/1 -> Switch/2
  Constant/1 -> Switch/1
  Constant2/1 -> Switch/3
  Switch/1 -> Product1/1, P/1, Product/1

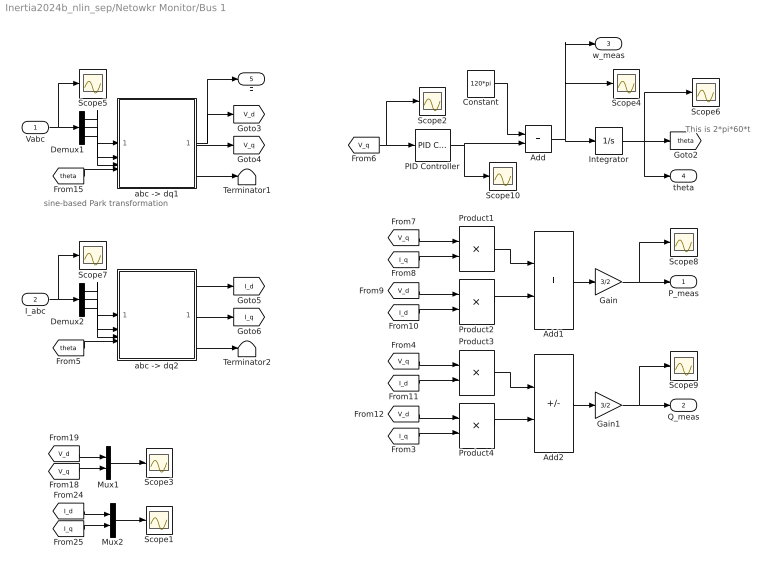
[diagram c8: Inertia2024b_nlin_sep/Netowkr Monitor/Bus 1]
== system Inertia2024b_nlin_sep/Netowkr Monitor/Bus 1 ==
  note: sine-based Park transformation
  note: This is 2*pi*60*t
  Vabc : Inport
  I_abc : Inport  Port=2
  Add : Sum
  Add1 : Sum
  Add2 : Sum  Inputs=+-
  Constant : Constant  Value=120*pi
  Demux1 : Demux  Outputs=3
  Demux2 : Demux  Outputs=3
  Gain : Gain  Gain=3/2
  Gain1 : Gain  Gain=3/2
  Integrator : Integrator  IgnoreLimit=on
  Mux1 : Mux  Inputs=2
  Mux2 : Mux  Inputs=2
  PID Controller : slpidlib/PID Controller  Controller=PI  Form=Parallel  TimeDomain=Continuous-time  UseExternalTs=off  SampleTime=-1  IntegratorMethod=Forward Euler  FilterMethod=Forward Euler  ControllerParametersSource=internal  P=K_prop_pll  I=K_int_pll  UseKiTs=off  D=0  UseExternalDerivativeSource=off  N=100  UseFilter=on  TunerSelectOption=Transfer Function Based (PID Tuner App)  InitialConditionSource=internal  InitialConditionForIntegrator=0  InitialConditionForFilter=0  DifferentiatorICPrevScaledInput=0  ExternalReset=none  IgnoreLimit=on  TrackingMode=off  Kt=1  LimitOutput=off  SatLimitsSource=internal  UpperSaturationLimit=inf  LowerSaturationLimit=-inf  LinearizeAsGain=on  AntiWindupMode=none  Kb=1  LimitIntegrator=off  UpperIntegratorSaturationLimit=inf  LowerIntegratorSaturationLimit=-inf  POutMin=[]  POutMax=[]  IOutMin=[]  IOutMax=[]  DOutMin=[]  DOutMax=[]  NOutMin=[]  NOutMax=[]  SumOutMin=[]  SumOutMax=[]  SaturationOutMin=[]  SaturationOutMax=[]  PParamMin=[]  PParamMax=[]  IParamMin=[]  IParamMax=[]  DParamMin=[]  DParamMax=[]  NParamMin=[]  NParamMax=[]  KbParamMin=[]  KbParamMax=[]  KtParamMin=[]  KtParamMax=[]  KbOutMin=[]  KbOutMax=[]  KtOutMin=[]  KtOutMax=[]  IntegratorOutMin=[]  IntegratorOutMax=[]  FilterOutMin=[]  FilterOutMax=[]  SumI1OutMin=[]  SumI1OutMax=[]  SumI2OutMin=[]  SumI2OutMax=[]  SumI3OutMin=[]  SumI3OutMax=[]  SumI4OutMin=[]  SumI4OutMax=[]  SumDOutMin=[]  SumDOutMax=[]  DifferentiatorOutMin=[]  DifferentiatorOutMax=[]  FilterDiffOutCoefMin=[]  FilterDiffOutCoefMax=[]  ReciprocalOutMin=[]  ReciprocalOutMax=[]  SumDenOutMin=[]  SumDenOutMax=[]  SumNumOutMin=[]  SumNumOutMax=[]  DivideOutMin=[]  DivideOutMax=[]  UdiffTsProdOutMin=[]  UdiffTsProdOutMax=[]  NTsProdOutMin=[]  NTsProdOutMax=[]  UintegralTsProdOutMin=[]  UintegralTsProdOutMax=[]  UngainTsProdOutMin=[]  UngainTsProdOutMax=[]  ClampingZeroOutDataTypeStr=Inherit: Inherit via back propagation  ClampingZeroOutMin=[]  ClampingZeroOutMax=[]  FilterDenConstantOutDataTypeStr=Inherit: Inherit via back propagation  FilterDenConstantOutMin=[]  FilterDenConstantOutMax=[]  PCopyOutDataTypeStr=Inherit: Inherit via back propagation  PCopyOutMin=[]  PCopyOutMax=[]  NCopyOutDataTypeStr=Inherit: Inherit via back propagation  NCopyOutMin=[]  NCopyOutMax=[]  IntegratorContinuousStateAttributes=''  IntegratorStateMustResolveToSignalObject=off  IntegratorRTWStateStorageClass=Auto  FilterContinuousStateAttributes=''  FilterStateMustResolveToSignalObject=off  FilterRTWStateStorageClass=Auto  ParallelPVariant=InternalParameters  IdealPVariant=Disabled  IVariant=InternalParameters  DVariant=Disabled  IntegratorVariant=Continuous  SatVariant=Disabled  AWVariant=Passthrough  PCopyVariant=Disabled  TRVariant=Disabled  FdbkBlocksVariant=Forward  IdealPFdbkVariant=Disabled  SatFdbkVariant=Disabled  DerivativeFilterVariant=Disabled  NVariant=Disabled  NCopyVariant=Disabled_SignalSpec  FilterICVariant=Disabled  IntegratorICVariant=InternalICs  ExternalResetVariant=Disabled  TRSumVariant=Passthrough  SumFdbkVariant=Disabled  SumVariant=Sum_PI  TsampFilterVariant=InternalTs  TsampNgainVariant=Passthrough  TsampIntegralVariant=Disabled_SignalSpec  ExternalSaturationOutDataTypeStr=Inherit: Same as second input  DerivativeSourceVariant=Disabled  PreIntVariant=InternalPreInt
  Product{1..4} (4 alike) : Product
  Scope{1..10} (10 alike) : Scope
  Terminator1 : Terminator
  Terminator2 : Terminator
  "abc -> dq1" : Subsystem
  "abc -> dq2" : Subsystem
  P_meas : Outport  VectorParamsAs1DForOutWhenUnconnected=off
  Q_meas : Outport  Port=2  VectorParamsAs1DForOutWhenUnconnected=off
  w_meas : Outport  Port=3  VectorParamsAs1DForOutWhenUnconnected=off
  theta : Outport  Port=4  VectorParamsAs1DForOutWhenUnconnected=off
  E : Outport  Port=5  VectorParamsAs1DForOutWhenUnconnected=off
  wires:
  Add/1 -> Integrator/1, w_meas/1, Scope4/1
  [V_q] -> Scope2/1, PID Controller/1
  PID Controller/1 -> Scope10/1, Add/2
  Constant/1 -> Add/1
  Demux1/2 -> "abc -> dq1"/2(b)
  Demux1/3 -> "abc -> dq1"/3(c)
  [theta] -> "abc -> dq1"/4(Theta)
  Vabc/1 -> Scope5/1, Demux1/1
  Demux1/1 -> "abc -> dq1"/1(a)
  "abc -> dq1"/3(0) -> Terminator1/1
  "abc -> dq1"/2(q) -> [V_q]
  Integrator/1 -> [theta], theta/1, Scope6/1
  Demux2/2 -> "abc -> dq2"/2(b)
  Demux2/3 -> "abc -> dq2"/3(c)
  [theta] -> "abc -> dq2"/4(Theta)
  I_abc/1 -> Scope7/1, Demux2/1
  Demux2/1 -> "abc -> dq2"/1(a)
  "abc -> dq2"/3(0) -> Terminator2/1
  "abc -> dq2"/2(q) -> [I_q]
  "abc -> dq2"/1(d) -> [I_d]
  [V_q] -> Product1/1
  [I_q] -> Product1/2
  Product1/1 -> Add1/1
  [V_d] -> Product2/1
  [I_d] -> Product2/2
  Product2/1 -> Add1/2
  Add1/1 -> Gain/1
  Gain/1 -> Scope8/1, P_meas/1
  [V_q] -> Product3/1
  [I_d] -> Product3/2
  Product3/1 -> Add2/1
  [V_d] -> Product4/1
  [I_q] -> Product4/2
  Product4/1 -> Add2/2
  Add2/1 -> Gain1/1
  Gain1/1 -> Scope9/1, Q_meas/1
  [V_d] -> Mux1/1
  [I_d] -> Mux2/1
  [I_q] -> Mux2/2
  [V_q] -> Mux1/2
  Mux1/1 -> Scope3/1
  Mux2/1 -> Scope1/1
  "abc -> dq1"/1(d) -> E/1, [V_d]

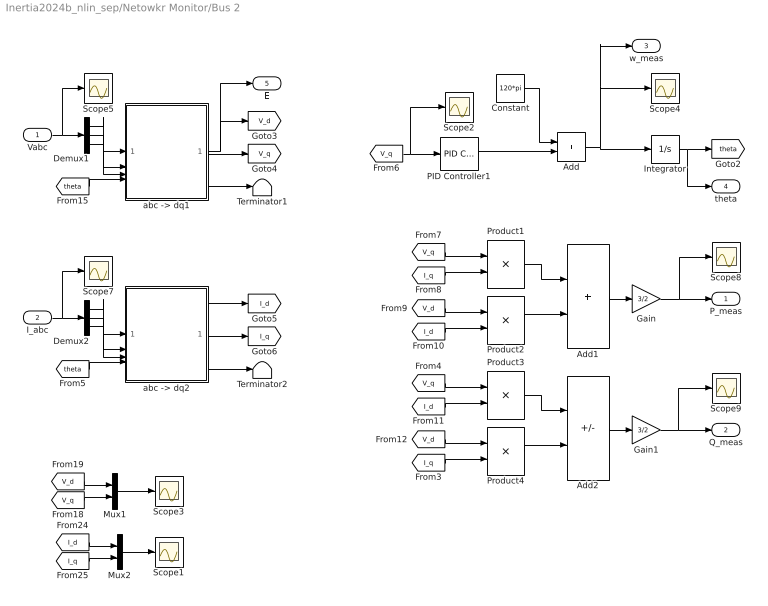
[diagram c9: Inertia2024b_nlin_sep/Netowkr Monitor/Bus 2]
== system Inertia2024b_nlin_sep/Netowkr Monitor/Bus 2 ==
  Vabc : Inport
  I_abc : Inport  Port=2
  Add : Sum
  Add1 : Sum
  Add2 : Sum  Inputs=+-
  Constant : Constant  Value=120*pi
  Demux1 : Demux  Outputs=3
  Demux2 : Demux  Outputs=3
  Gain : Gain  Gain=3/2
  Gain1 : Gain  Gain=3/2
  Integrator : Integrator  IgnoreLimit=on
  Mux1 : Mux  Inputs=2
  Mux2 : Mux  Inputs=2
  PID Controller1 : slpidlib/PID Controller  Controller=PI  Form=Parallel  TimeDomain=Continuous-time  UseExternalTs=off  SampleTime=-1  IntegratorMethod=Forward Euler  FilterMethod=Forward Euler  ControllerParametersSource=internal  P=K_prop_pll  I=K_int_pll  UseKiTs=off  D=0  UseExternalDerivativeSource=off  N=100  UseFilter=on  TunerSelectOption=Transfer Function Based (PID Tuner App)  InitialConditionSource=internal  InitialConditionForIntegrator=0  InitialConditionForFilter=0  DifferentiatorICPrevScaledInput=0  ExternalReset=none  IgnoreLimit=on  TrackingMode=off  Kt=1  LimitOutput=off  SatLimitsSource=internal  UpperSaturationLimit=inf  LowerSaturationLimit=-inf  LinearizeAsGain=on  AntiWindupMode=none  Kb=1  LimitIntegrator=off  UpperIntegratorSaturationLimit=inf  LowerIntegratorSaturationLimit=-inf  POutMin=[]  POutMax=[]  IOutMin=[]  IOutMax=[]  DOutMin=[]  DOutMax=[]  NOutMin=[]  NOutMax=[]  SumOutMin=[]  SumOutMax=[]  SaturationOutMin=[]  SaturationOutMax=[]  PParamMin=[]  PParamMax=[]  IParamMin=[]  IParamMax=[]  DParamMin=[]  DParamMax=[]  NParamMin=[]  NParamMax=[]  KbParamMin=[]  KbParamMax=[]  KtParamMin=[]  KtParamMax=[]  KbOutMin=[]  KbOutMax=[]  KtOutMin=[]  KtOutMax=[]  IntegratorOutMin=[]  IntegratorOutMax=[]  FilterOutMin=[]  FilterOutMax=[]  SumI1OutMin=[]  SumI1OutMax=[]  SumI2OutMin=[]  SumI2OutMax=[]  SumI3OutMin=[]  SumI3OutMax=[]  SumI4OutMin=[]  SumI4OutMax=[]  SumDOutMin=[]  SumDOutMax=[]  DifferentiatorOutMin=[]  DifferentiatorOutMax=[]  FilterDiffOutCoefMin=[]  FilterDiffOutCoefMax=[]  ReciprocalOutMin=[]  ReciprocalOutMax=[]  SumDenOutMin=[]  SumDenOutMax=[]  SumNumOutMin=[]  SumNumOutMax=[]  DivideOutMin=[]  DivideOutMax=[]  UdiffTsProdOutMin=[]  UdiffTsProdOutMax=[]  NTsProdOutMin=[]  NTsProdOutMax=[]  UintegralTsProdOutMin=[]  UintegralTsProdOutMax=[]  UngainTsProdOutMin=[]  UngainTsProdOutMax=[]  ClampingZeroOutDataTypeStr=Inherit: Inherit via back propagation  ClampingZeroOutMin=[]  ClampingZeroOutMax=[]  FilterDenConstantOutDataTypeStr=Inherit: Inherit via back propagation  FilterDenConstantOutMin=[]  FilterDenConstantOutMax=[]  PCopyOutDataTypeStr=Inherit: Inherit via back propagation  PCopyOutMin=[]  PCopyOutMax=[]  NCopyOutDataTypeStr=Inherit: Inherit via back propagation  NCopyOutMin=[]  NCopyOutMax=[]  IntegratorContinuousStateAttributes=''  IntegratorStateMustResolveToSignalObject=off  IntegratorRTWStateStorageClass=Auto  FilterContinuousStateAttributes=''  FilterStateMustResolveToSignalObject=off  FilterRTWStateStorageClass=Auto  ParallelPVariant=InternalParameters  IdealPVariant=Disabled  IVariant=InternalParameters  DVariant=Disabled  IntegratorVariant=Continuous  SatVariant=Disabled  AWVariant=Passthrough  PCopyVariant=Disabled  TRVariant=Disabled  FdbkBlocksVariant=Forward  IdealPFdbkVariant=Disabled  SatFdbkVariant=Disabled  DerivativeFilterVariant=Disabled  NVariant=Disabled  NCopyVariant=Disabled_SignalSpec  FilterICVariant=Disabled  IntegratorICVariant=InternalICs  ExternalResetVariant=Disabled  TRSumVariant=Passthrough  SumFdbkVariant=Disabled  SumVariant=Sum_PI  TsampFilterVariant=InternalTs  TsampNgainVariant=Passthrough  TsampIntegralVariant=Disabled_SignalSpec  ExternalSaturationOutDataTypeStr=Inherit: Same as second input  DerivativeSourceVariant=Disabled  PreIntVariant=InternalPreInt
  Product{1..4} (4 alike) : Product
  Scope{1..5,7..9} (8 alike) : Scope
  Terminator1 : Terminator
  Terminator2 : Terminator
  "abc -> dq1" : Subsystem
  "abc -> dq2" : Subsystem
  P_meas : Outport  VectorParamsAs1DForOutWhenUnconnected=off
  Q_meas : Outport  Port=2  VectorParamsAs1DForOutWhenUnconnected=off
  w_meas : Outport  Port=3  VectorParamsAs1DForOutWhenUnconnected=off
  theta : Outport  Port=4  VectorParamsAs1DForOutWhenUnconnected=off
  E : Outport  Port=5  VectorParamsAs1DForOutWhenUnconnected=off
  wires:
  Add/1 -> Integrator/1, w_meas/1, Scope4/1
  [V_q] -> PID Controller1/1, Scope2/1
  PID Controller1/1 -> Add/2
  Constant/1 -> Add/1
  Demux1/2 -> "abc -> dq1"/2(b)
  Demux1/3 -> "abc -> dq1"/3(c)
  [theta] -> "abc -> dq1"/4(Theta)
  Vabc/1 -> Scope5/1, Demux1/1
  Demux1/1 -> "abc -> dq1"/1(a)
  "abc -> dq1"/3(0) -> Terminator1/1
  "abc -> dq1"/2(q) -> [V_q]
  Integrator/1 -> theta/1, [theta]
  Demux2/2 -> "abc -> dq2"/2(b)
  Demux2/3 -> "abc -> dq2"/3(c)
  [theta] -> "abc -> dq2"/4(Theta)
  I_abc/1 -> Scope7/1, Demux2/1
  Demux2/1 -> "abc -> dq2"/1(a)
  "abc -> dq2"/3(0) -> Terminator2/1
  "abc -> dq2"/2(q) -> [I_q]
  "abc -> dq2"/1(d) -> [I_d]
  [V_q] -> Product1/1
  [I_q] -> Product1/2
  Product1/1 -> Add1/1
  [V_d] -> Product2/1
  [I_d] -> Product2/2
  Product2/1 -> Add1/2
  Add1/1 -> Gain/1
  Gain/1 -> Scope8/1, P_meas/1
  [V_q] -> Product3/1
  [I_d] -> Product3/2
  Product3/1 -> Add2/1
  [V_d] -> Product4/1
  [I_q] -> Product4/2
  Product4/1 -> Add2/2
  Add2/1 -> Gain1/1
  Gain1/1 -> Scope9/1, Q_meas/1
  [V_d] -> Mux1/1
  [I_d] -> Mux2/1
  [I_q] -> Mux2/2
  [V_q] -> Mux1/2
  Mux1/1 -> Scope3/1
  Mux2/1 -> Scope1/1
  "abc -> dq1"/1(d) -> E/1, [V_d]

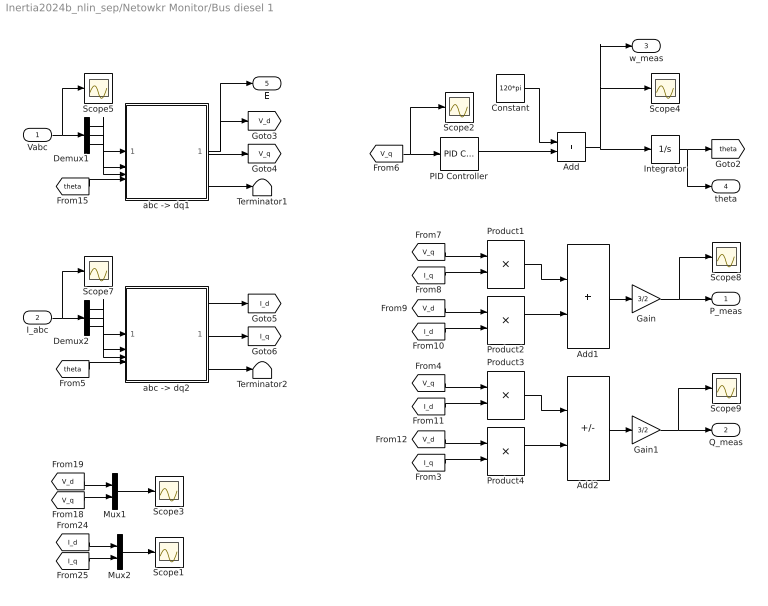
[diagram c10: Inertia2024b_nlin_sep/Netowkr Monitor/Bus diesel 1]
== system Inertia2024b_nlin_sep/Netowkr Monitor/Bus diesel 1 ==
  Vabc : Inport
  I_abc : Inport  Port=2
  Add : Sum
  Add1 : Sum
  Add2 : Sum  Inputs=+-
  Constant : Constant  Value=120*pi
  Demux1 : Demux  Outputs=3
  Demux2 : Demux  Outputs=3
  Gain : Gain  Gain=3/2
  Gain1 : Gain  Gain=3/2
  Integrator : Integrator  IgnoreLimit=on
  Mux1 : Mux  Inputs=2
  Mux2 : Mux  Inputs=2
  PID Controller : slpidlib/PID Controller  Controller=PI  Form=Parallel  TimeDomain=Continuous-time  UseExternalTs=off  SampleTime=-1  IntegratorMethod=Forward Euler  FilterMethod=Forward Euler  ControllerParametersSource=internal  P=K_prop_pll  I=K_int_pll  UseKiTs=off  D=0  UseExternalDerivativeSource=off  N=100  UseFilter=on  TunerSelectOption=Transfer Function Based (PID Tuner App)  InitialConditionSource=internal  InitialConditionForIntegrator=0  InitialConditionForFilter=0  DifferentiatorICPrevScaledInput=0  ExternalReset=none  IgnoreLimit=on  TrackingMode=off  Kt=1  LimitOutput=off  SatLimitsSource=internal  UpperSaturationLimit=inf  LowerSaturationLimit=-inf  LinearizeAsGain=on  AntiWindupMode=none  Kb=1  LimitIntegrator=off  UpperIntegratorSaturationLimit=inf  LowerIntegratorSaturationLimit=-inf  POutMin=[]  POutMax=[]  IOutMin=[]  IOutMax=[]  DOutMin=[]  DOutMax=[]  NOutMin=[]  NOutMax=[]  SumOutMin=[]  SumOutMax=[]  SaturationOutMin=[]  SaturationOutMax=[]  PParamMin=[]  PParamMax=[]  IParamMin=[]  IParamMax=[]  DParamMin=[]  DParamMax=[]  NParamMin=[]  NParamMax=[]  KbParamMin=[]  KbParamMax=[]  KtParamMin=[]  KtParamMax=[]  KbOutMin=[]  KbOutMax=[]  KtOutMin=[]  KtOutMax=[]  IntegratorOutMin=[]  IntegratorOutMax=[]  FilterOutMin=[]  FilterOutMax=[]  SumI1OutMin=[]  SumI1OutMax=[]  SumI2OutMin=[]  SumI2OutMax=[]  SumI3OutMin=[]  SumI3OutMax=[]  SumI4OutMin=[]  SumI4OutMax=[]  SumDOutMin=[]  SumDOutMax=[]  DifferentiatorOutMin=[]  DifferentiatorOutMax=[]  FilterDiffOutCoefMin=[]  FilterDiffOutCoefMax=[]  ReciprocalOutMin=[]  ReciprocalOutMax=[]  SumDenOutMin=[]  SumDenOutMax=[]  SumNumOutMin=[]  SumNumOutMax=[]  DivideOutMin=[]  DivideOutMax=[]  UdiffTsProdOutMin=[]  UdiffTsProdOutMax=[]  NTsProdOutMin=[]  NTsProdOutMax=[]  UintegralTsProdOutMin=[]  UintegralTsProdOutMax=[]  UngainTsProdOutMin=[]  UngainTsProdOutMax=[]  ClampingZeroOutDataTypeStr=Inherit: Inherit via back propagation  ClampingZeroOutMin=[]  ClampingZeroOutMax=[]  FilterDenConstantOutDataTypeStr=Inherit: Inherit via back propagation  FilterDenConstantOutMin=[]  FilterDenConstantOutMax=[]  PCopyOutDataTypeStr=Inherit: Inherit via back propagation  PCopyOutMin=[]  PCopyOutMax=[]  NCopyOutDataTypeStr=Inherit: Inherit via back propagation  NCopyOutMin=[]  NCopyOutMax=[]  IntegratorContinuousStateAttributes=''  IntegratorStateMustResolveToSignalObject=off  IntegratorRTWStateStorageClass=Auto  FilterContinuousStateAttributes=''  FilterStateMustResolveToSignalObject=off  FilterRTWStateStorageClass=Auto  ParallelPVariant=InternalParameters  IdealPVariant=Disabled  IVariant=InternalParameters  DVariant=Disabled  IntegratorVariant=Continuous  SatVariant=Disabled  AWVariant=Passthrough  PCopyVariant=Disabled  TRVariant=Disabled  FdbkBlocksVariant=Forward  IdealPFdbkVariant=Disabled  SatFdbkVariant=Disabled  DerivativeFilterVariant=Disabled  NVariant=Disabled  NCopyVariant=Disabled_SignalSpec  FilterICVariant=Disabled  IntegratorICVariant=InternalICs  ExternalResetVariant=Disabled  TRSumVariant=Passthrough  SumFdbkVariant=Disabled  SumVariant=Sum_PI  TsampFilterVariant=InternalTs  TsampNgainVariant=Passthrough  TsampIntegralVariant=Disabled_SignalSpec  ExternalSaturationOutDataTypeStr=Inherit: Same as second input  DerivativeSourceVariant=Disabled  PreIntVariant=InternalPreInt
  Product{1..4} (4 alike) : Product
  Scope{1..5,7..9} (8 alike) : Scope
  Terminator1 : Terminator
  Terminator2 : Terminator
  "abc -> dq1" : Subsystem
  "abc -> dq2" : Subsystem
  P_meas : Outport  VectorParamsAs1DForOutWhenUnconnected=off
  Q_meas : Outport  Port=2  VectorParamsAs1DForOutWhenUnconnected=off
  w_meas : Outport  Port=3  VectorParamsAs1DForOutWhenUnconnected=off
  theta : Outport  Port=4  VectorParamsAs1DForOutWhenUnconnected=off
  E : Outport  Port=5  VectorParamsAs1DForOutWhenUnconnected=off
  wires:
  Add/1 -> Integrator/1, w_meas/1, Scope4/1
  [V_q] -> Scope2/1, PID Controller/1
  PID Controller/1 -> Add/2
  Constant/1 -> Add/1
  Demux1/2 -> "abc -> dq1"/2(b)
  Demux1/3 -> "abc -> dq1"/3(c)
  [theta] -> "abc -> dq1"/4(Theta)
  Vabc/1 -> Scope5/1, Demux1/1
  Demux1/1 -> "abc -> dq1"/1(a)
  "abc -> dq1"/3(0) -> Terminator1/1
  "abc -> dq1"/2(q) -> [V_q]
  Integrator/1 -> theta/1, [theta]
  Demux2/2 -> "abc -> dq2"/2(b)
  Demux2/3 -> "abc -> dq2"/3(c)
  [theta] -> "abc -> dq2"/4(Theta)
  I_abc/1 -> Scope7/1, Demux2/1
  Demux2/1 -> "abc -> dq2"/1(a)
  "abc -> dq2"/3(0) -> Terminator2/1
  "abc -> dq2"/2(q) -> [I_q]
  "abc -> dq2"/1(d) -> [I_d]
  [V_q] -> Product1/1
  [I_q] -> Product1/2
  Product1/1 -> Add1/1
  [V_d] -> Product2/1
  [I_d] -> Product2/2
  Product2/1 -> Add1/2
  Add1/1 -> Gain/1
  Gain/1 -> Scope8/1, P_meas/1
  [V_q] -> Product3/1
  [I_d] -> Product3/2
  Product3/1 -> Add2/1
  [V_d] -> Product4/1
  [I_q] -> Product4/2
  Product4/1 -> Add2/2
  Add2/1 -> Gain1/1
  Gain1/1 -> Scope9/1, Q_meas/1
  [V_d] -> Mux1/1
  [I_d] -> Mux2/1
  [I_q] -> Mux2/2
  [V_q] -> Mux1/2
  Mux1/1 -> Scope3/1
  Mux2/1 -> Scope1/1
  "abc -> dq1"/1(d) -> E/1, [V_d]
